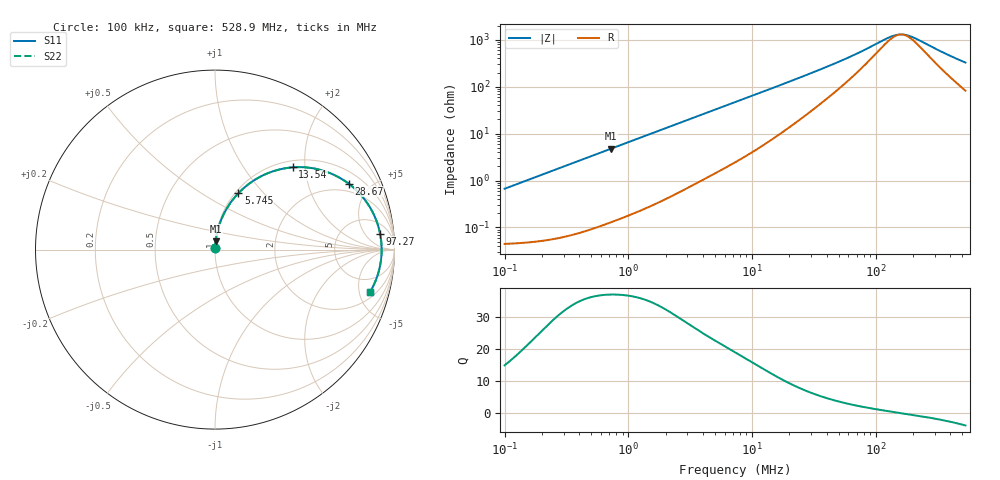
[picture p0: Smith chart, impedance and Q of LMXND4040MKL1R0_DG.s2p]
! LMXND4040MKL1R0_DG  S-PARAMETER MODEL  ( General Type )
! Model Generated by TAIYO YUDEN Corporation (https://www.yuden.co.jp/en/)
! Version 1.0
! TAIYO YUDEN Control No. 191023NI43SB-FBB
! Copyright(c) 2019 TAIYO YUDEN CO.,LTD. All Rights Reserved.
! Product Description (link to TY-COMPAS)
! https://ds.yuden.co.jp/TYCOMPAS/or/detail?pn=LMXND4040MKL1R0NDG&u=M
! Products Name : Inductors
! Characteristics :
!  Inductance : 1.0 uH , SRF(min) : 100 MHz , DC Resistance(max) : 0.0504 Ohm
!  Rated Current : Saturation :2800 mA , Temp Rise : 2200 mA (40 degC)
!  Case Size : 4.0 x 4.0 / 0.157 x 0.157 [mm/inch] , Thickness : 1.2 / 0.047 [mm/inch]
!  (Conditions: Temperature = 25 degC , DC Bias Current/Voltage = 0A / 0V)
! External Node Assignments :
!  1  o---GGG---o  2
! GND o---------o GND
! Frequency Range : 0.1MHz  -  528.887669MHz  [ 402 STEP ]
# MHz S RI R 50
! Freq[MHz].  S11 Real  S11 Imag  S21 Real  S21 Imag  S12 Real  S12 Imag  S22 Real  S22 Imag
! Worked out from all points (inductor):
!   401 points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, 100 kHz to 528.9 MHz, reference 50 ohm
!   read as one part in series: L = 1.06 uH near 104.4 kHz
!   highest Q = 37.1 at 718.4 kHz (marker M1), where L = 1.05 uH
!   self-resonance near 160.1 MHz
!   S11 on the Smith chart (normalised r, x): 100 kHz: 1.00, +0.01; 5.745 MHz: 1.03, +0.74; 13.54 MHz: 1.13, +1.72; 28.67 MHz: 1.55, +3.67; 97.27 MHz: 10, +12; 528.9 MHz: 2.65, -6.33
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0.1  0.000489 0.00665  0.9995 -0.00665  0.9995 -0.00665  0.000489 0.00665
0.420401  0.00156 0.0278  0.9984 -0.0278  0.9984 -0.0278  0.00156 0.0278
0.718412  0.0035 0.0471  0.9965 -0.0471  0.9965 -0.0471  0.0035 0.0471
1.767367  0.0164 0.113  0.9836 -0.113  0.9836 -0.113  0.0164 0.113
3.434689  0.0541 0.2082  0.9459 -0.2082  0.9459 -0.2082  0.0541 0.2082
5.744989  0.1308 0.3146  0.8692 -0.3146  0.8692 -0.3146  0.1308 0.3146
7.430023  0.1967 0.3719  0.8033 -0.3719  0.8033 -0.3719  0.1967 0.3719
10.24746  0.3107 0.432  0.6893 -0.432  0.6893 -0.432  0.3107 0.432
13.54021  0.4328 0.4583  0.5672 -0.4583  0.5672 -0.4583  0.4328 0.4583
19.0792  0.59 0.4432  0.41 -0.4432  0.41 -0.4432  0.59 0.4432
28.66948  0.745 0.3672  0.255 -0.3672  0.255 -0.3672  0.745 0.3672
30.5735  0.7644 0.3518  0.2356 -0.3518  0.2356 -0.3518  0.7644 0.3518
39.54085  0.8274 0.2873  0.1726 -0.2873  0.1726 -0.2873  0.8274 0.2873
51.13837  0.8703 0.2236  0.1297 -0.2236  0.1297 -0.2236  0.8703 0.2236
70.52986  0.9029 0.1511  0.0971 -0.1511  0.0971 -0.1511  0.9029 0.1511
97.27454  0.9201 0.0874  0.0799 -0.0874  0.0799 -0.0874  0.9201 0.0874
128.5312  0.9269 0.0375  0.0731 -0.0375  0.0731 -0.0375  0.9269 0.0375
155.8778  0.9285 0.00452  0.0715 -0.00452  0.0715 -0.00452  0.9285 0.00452
185.034  0.9279 -0.0247  0.0721 0.0247  0.0721 0.0247  0.9279 -0.0247
214.9861  0.9258 -0.0507  0.0742 0.0507  0.0742 0.0507  0.9258 -0.0507
367.3842  0.9024 -0.1536  0.0976 0.1536  0.0976 0.1536  0.9024 -0.1536
528.8877  0.8634 -0.2371  0.1366 0.2371  0.1366 0.2371  0.8634 -0.2371
